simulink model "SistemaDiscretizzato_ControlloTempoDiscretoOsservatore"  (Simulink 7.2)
settings: Solver=ode3  StartTime=0.0  StopTime=10.0  FixedStep=Ts  RelTol=1e-3
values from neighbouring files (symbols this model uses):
  L = -acker(Az',Cz',[0 0 0])'    [TSC130625ProvaMatlab.m]
  X0 = [0.5 2 -0.5]'    [TSC130625ProvaMatlab.m]
undefined symbols (not defined in the file or in its folder): Az, Bz, Cz, K
libraries: simulink x2

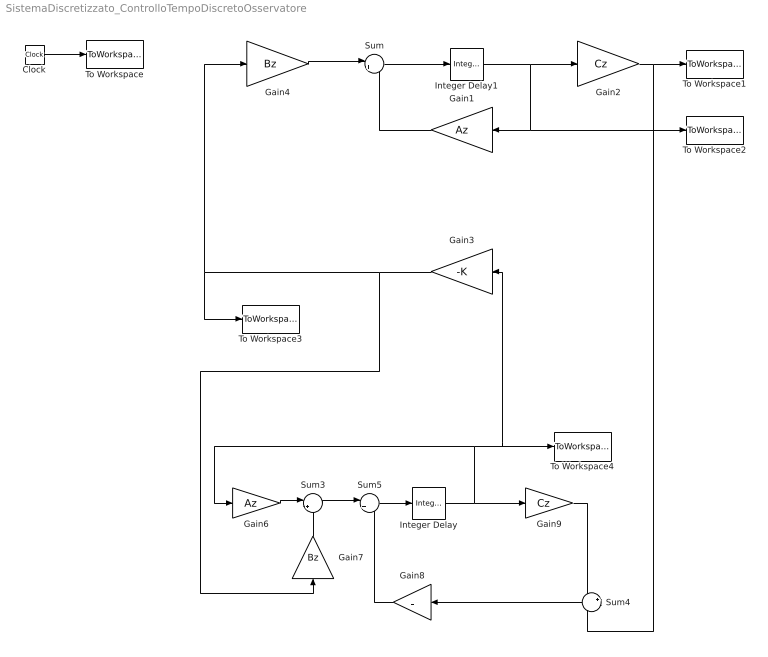
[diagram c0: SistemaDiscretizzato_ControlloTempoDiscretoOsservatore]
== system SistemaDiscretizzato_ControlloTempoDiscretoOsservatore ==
  Clock : Clock
  Gain1 : Gain  Orientation=left  Gain=Az  Multiplication=Matrix(K*u)  ParameterDataType=sfix(16)  ParameterScaling=2^0  OutDataType=sfix(16)  OutScaling=2^0
  Gain2 : Gain  Gain=Cz  Multiplication=Matrix(K*u)  ParameterDataType=sfix(16)  ParameterScaling=2^0  OutDataType=sfix(16)  OutScaling=2^0
  Gain3 : Gain  Orientation=left  Gain=-K  Multiplication=Matrix(K*u)  ParameterDataType=sfix(16)  ParameterScaling=2^0  OutDataType=sfix(16)  OutScaling=2^0
  Gain4 : Gain  Gain=Bz  Multiplication=Matrix(K*u)  ParameterDataType=sfix(16)  ParameterScaling=2^0  OutDataType=sfix(16)  OutScaling=2^0
  Gain6 : Gain  Gain=Az  Multiplication=Matrix(K*u)  ParameterDataType=sfix(16)  ParameterScaling=2^0  OutDataType=sfix(16)  OutScaling=2^0
  Gain7 : Gain  Orientation=up  Gain=Bz  Multiplication=Matrix(K*u)  ParameterDataType=sfix(16)  ParameterScaling=2^0  OutDataType=sfix(16)  OutScaling=2^0
  Gain8 : Gain  Orientation=left  Gain=L  Multiplication=Matrix(K*u)  ParameterDataType=sfix(16)  ParameterScaling=2^0  OutDataType=sfix(16)  OutScaling=2^0
  Gain9 : Gain  Gain=Cz  Multiplication=Matrix(K*u)  ParameterDataType=sfix(16)  ParameterScaling=2^0  OutDataType=sfix(16)  OutScaling=2^0
  Integer Delay : simulink/Discrete/Integer Delay  vinit=[0 0 0]'  samptime=Ts  NumDelays=1
  Integer Delay1 : simulink/Discrete/Integer Delay  vinit=X0  samptime=Ts  NumDelays=1
  Sum : Sum  Inputs=|++  OutDataType=sfix(16)  OutScaling=2^0
  Sum3 : Sum  Inputs=|++  OutDataType=sfix(16)  OutScaling=2^0
  Sum4 : Sum  Orientation=left  Inputs=+-  OutDataType=sfix(16)  OutScaling=2^0
  Sum5 : Sum  Inputs=|++  OutDataType=sfix(16)  OutScaling=2^0
  To Workspace : ToWorkspace  VariableName=time  SampleTime=-1  SaveFormat=Array
  To Workspace1 : ToWorkspace  VariableName=y  SampleTime=-1  SaveFormat=Array
  To Workspace2 : ToWorkspace  VariableName=X  SampleTime=-1  SaveFormat=Array
  To Workspace3 : ToWorkspace  VariableName=ud  SampleTime=-1  SaveFormat=Array
  To Workspace4 : ToWorkspace  VariableName=Xs  SampleTime=-1  SaveFormat=Array
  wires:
  Gain1/1 -> Sum/2
  Sum/1 -> Integer Delay1/1
  Integer Delay1/1 -> Gain2/1, Gain1/1, To Workspace2/1
  Gain2/1 -> To Workspace1/1, Sum4/2
  Gain4/1 -> Sum/1
  Gain3/1 -> Gain7/1, Gain4/1, To Workspace3/1
  Clock/1 -> To Workspace/1
  Gain6/1 -> Sum3/1
  Integer Delay/1 -> Gain9/1, Gain6/1, Gain3/1, To Workspace4/1
  Gain7/1 -> Sum3/2
  Sum4/1 -> Gain8/1
  Gain9/1 -> Sum4/1
  Gain8/1 -> Sum5/2
  Sum3/1 -> Sum5/1
  Sum5/1 -> Integer Delay/1
